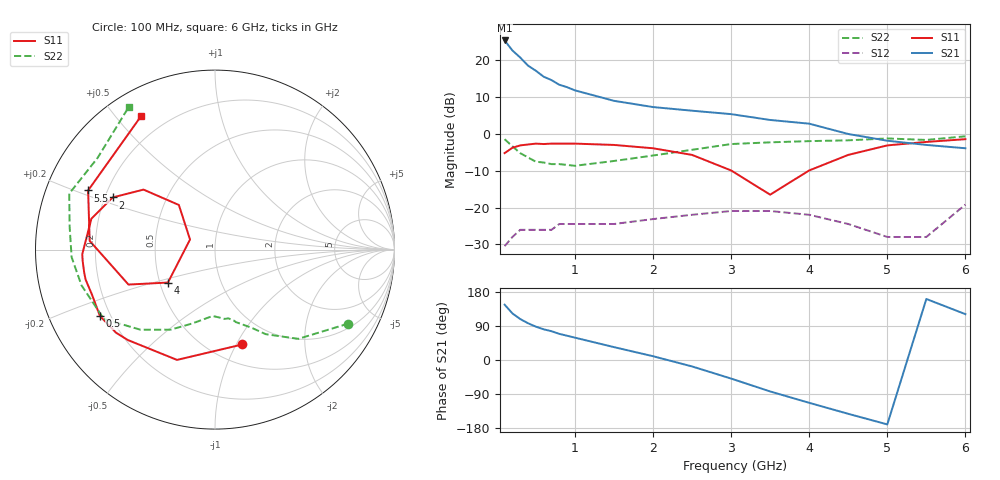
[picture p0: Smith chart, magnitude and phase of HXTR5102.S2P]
! HXTR-5102 Common Emitter
! Vce=18V  Ic=110mA
# ghz s ma r 50
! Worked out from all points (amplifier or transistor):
!   20 points, 100 MHz to 6 GHz, reference 50 ohm
!   highest |S21| = 25.4 dB at 100 MHz (marker M1)
!   |S21| within 3 dB of that: start of sweep to 214.6 MHz
!   unconditionally stable (mu >= 1): 1.491 GHz to 5.66 GHz
!   at 400 MHz: K = 0.37, MSG = 22.3 dB, |S12| = -26.0 dB
!   at 1.5 GHz: K = 1.01, MAG = 16.2 dB, |S12| = -24.4 dB
!   at 6 GHz: K = 0.48, MSG = 7.6 dB, |S12| = -19.2 dB
!   S11 on the Smith chart (normalised r, x): 100 MHz: 0.70, -1.06; 500 MHz: 0.16, -0.26; 2 GHz: 0.23, +0.23; 4 GHz: 0.55, -0.23; 5.5 GHz: 0.13, +0.22; 6 GHz: 0.11, +0.58
0.1  0.55 -74.0  18.6 146.0  0.03 56.0  0.85 -29.0
0.2  0.65 -109.0  13.6 123.0  0.04 39.0  0.68 -47.0
0.3  0.7 -134.0  10.9 108.0  0.05 28.0  0.55 -59.0
0.4  0.72 -140.0  8.47 97.0  0.05 21.0  0.48 -65.0
0.5  0.74 -150.0  7.22 88.0  0.05 17.0  0.42 -74.0
0.6  0.73 -160.0  5.99 81.0  0.05 13.0  0.41 -75.0
0.7  0.74 -167.0  5.39 76.0  0.05 11.0  0.39 -79.0
0.8  0.74 -170.0  4.66 69.0  0.06 8.0  0.39 -82.0
0.9  0.74 -175.0  4.32 64.0  0.06 8.0  0.38 -86.0
1  0.74 -178.0  3.91 59.0  0.06 7.0  0.37 -92.0
1.5  0.71 166.0  2.82 34.0  0.06 -2.0  0.43 -107.0
2  0.64 153.0  2.32 10.0  0.07 -8.0  0.51 -119.0
2.5  0.52 140.0  2.07 -17.0  0.08 -22.0  0.61 -133.0
3  0.32 129.0  1.86 -49.0  0.09 -42.0  0.73 -148.0
3.5  0.15 158.0  1.55 -83.0  0.09 -67.0  0.77 -165.0
4  0.32 -145.0  1.38 -113.0  0.08 -98.0  0.8 -177.0
4.5  0.52 -158.0  1 -142.0  0.06 132.0  0.82 171.0
5  0.7 176.0  0.81 -170.0  0.04 50.0  0.87 159.0
5.5  0.78 155.0  0.71 161.0  0.04 85.0  0.83 142.0
6  0.85 119.0  0.64 121.0  0.11 16.0  0.93 121.0
